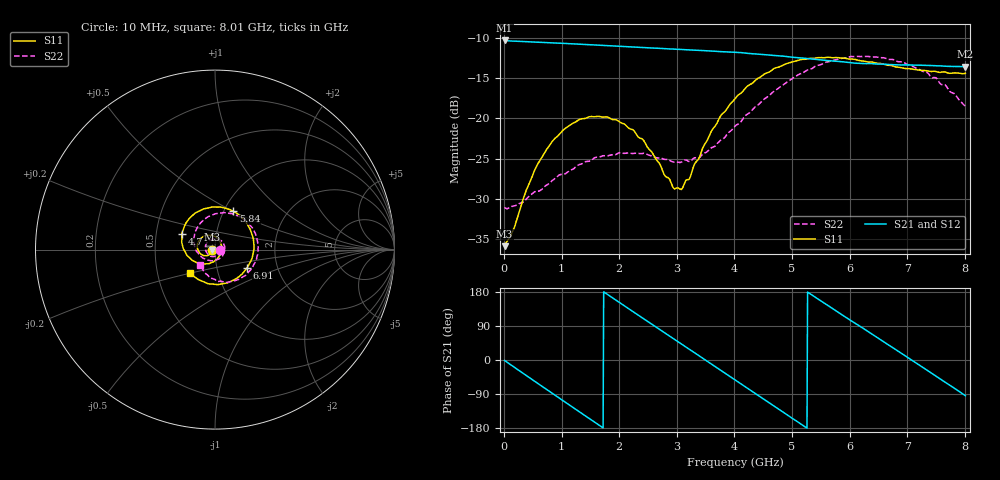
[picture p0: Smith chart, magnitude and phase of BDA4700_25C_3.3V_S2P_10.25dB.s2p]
!Agilent Technologies,E5071B,MY42404982,A.09.10
!Date: Mon Oct 20 18:07:19 2025
!Data & Calibration Information:
!Freq	S11:SOLT2(ON)	S21:SOLT2(ON)	S12:SOLT2(ON)	S22:SOLT2(ON)
# Hz S RI R 50
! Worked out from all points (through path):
!   801 points, 10 MHz to 8.01 GHz, reference 50 ohm
!   highest |S21| = -10.36 dB at 10 MHz (marker M1); lowest = -13.6 dB at 8 GHz (marker M2)
!   group delay of S21, straight-line fit = 282 ps
!   lowest |S11| = -35.9 dB at 10 MHz (marker M3), VSWR 1.03, Z = 48.4 - j0.12 ohm
!   |S11| at or under -10 dB: start of sweep to end of sweep
!   |S22| runs from -31.2 to -12.3 dB; largest |S21 - S12| = 0.0034
!   S11 on the Smith chart (normalised r, x): 10 MHz: 0.97, -0.00; 4.7 GHz: 0.68, +0.12; 5.84 GHz: 1.11, +0.50; 6.91 GHz: 1.39, -0.30; 8.01 GHz: 0.74, -0.20
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1e7  -0.0161 -0.00123  0.3034 -0.00667  0.3033 -0.00692  0.028 -0.0014
3.3e8  -0.0231 -0.0212  0.2446 -0.1716  0.2445 -0.1716  0.0225 -0.0201
7.2e8  -0.0521 -0.0343  0.0726 -0.2854  0.0728 -0.2854  -0.00216 -0.038
1.02e9  -0.0808 -0.023  -0.0843 -0.2786  -0.0842 -0.2787  -0.0296 -0.0338
1.35e9  -0.0987 0.00961  -0.2232 -0.1809  -0.2232 -0.1811  -0.0519 -0.00509
1.93e9  -0.0648 0.0735  -0.262 0.0991  -0.262 0.0992  -0.025 0.0538
2.32e9  -0.0129 0.0762  -0.1353 0.2397  -0.1352 0.2397  0.022 0.0565
2.68e9  0.0275 0.0459  0.0342 0.2691  0.0338 0.269  0.0523 0.022
2.94e9  0.0362 0.00769  0.1486 0.2234  0.1484 0.2228  0.0524 -0.0111
3.08e9  0.0332 -0.0144  0.1985 0.1782  0.1967 0.1794  0.045 -0.0291
3.53e9  -0.017 -0.0711  0.2612 -0.0165  0.2613 -0.0168  -0.00822 -0.0617
4.01e9  -0.114 -0.0664  0.1557 -0.2034  0.1561 -0.203  -0.0812 -0.0366
4.36e9  -0.1712 -0.00436  0.00764 -0.2503  0.00766 -0.2511  -0.1154 0.0228
4.7e9  -0.1854 0.0861  -0.1335 -0.2049  -0.1327 -0.2057  -0.1099 0.099
5.35e9  -0.0577 0.2281  -0.2301 0.036  -0.2302 0.0346  0.0247 0.202
5.84e9  0.1024 0.2129  -0.1197 0.1897  -0.1191 0.1895  0.169 0.1619
6.28e9  0.1998 0.1028  0.0404 0.2143  0.0433 0.2128  0.2386 0.0376
6.68e9  0.21 -0.0339  0.1667 0.1363  0.1671 0.1361  0.2157 -0.0846
6.91e9  0.1769 -0.1036  0.205 0.0611  0.2051 0.0602  0.1726 -0.1419
7.46e9  0.0208 -0.1944  0.1656 -0.1321  0.1655 -0.1324  0.0192 -0.1775
8e9  -0.1352 -0.1325  -0.0117 -0.2084  -0.0113 -0.2086  -0.0811 -0.0876
8.01e9  -0.1377 -0.1307  -0.0157 -0.2082  -0.0148 -0.2082  -0.0822 -0.0849
